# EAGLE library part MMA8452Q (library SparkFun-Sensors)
NXP MMA8452Q 3-Axis Digital Accelerometer The MMA8452Q is a smart low-power, three-axis, capacitive MEMS accelerometer with 12 bits of resolution. This accelerometer is packed with embedded functions with flexible user programmable options, configurable to two interrupt pins. Supply Voltage: 1.6-3.6V Range: +/- 2g, 4g, 8g Interface: I2C, 12-bit and 8-bit ODR: 1.56 Hz - 800 Hz Package: QFN-16 Datasheet SparkFun Products SparkFun Triple Axis Accelerometer Breakout - MMA8452Q (SEN-12756) SparkFun RedBot Sensor - Accelerometer (SEN-12589)
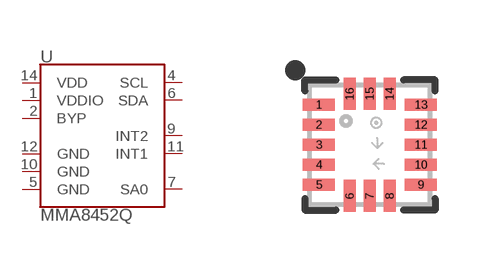
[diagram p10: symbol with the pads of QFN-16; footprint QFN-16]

Designator prefix U

## MMA8452Q (PROD_ID: IC-10769)  [QFN-16]
1  VDDIO
2  BYP
4  SCL
5  GND
6  SDA
7  SA0
9  INT2
10  GND
11  INT1
12  GND
14  VDD

## Footprint QFN-16 (pad centres in mm)
16-Pin Quad Flat No-Lead (QFN) (3 x 3 mm) Datasheet. Layout based on app note AN4077 Specifications: Pin Count: 16 Dimensions: 3.0 x 3.0 x 1.0 mm Pitch: 0.5 mm Devices Using: MMA8452Q
smd 0.8 x 0.3: 1 -1.275,1; 2 -1.275,0.5; 3 -1.275,0; 4 -1.275,-0.5; 5 -1.275,-1; 9 1.275,-1; 10 1.275,-0.5; 11 1.275,0; 12 1.275,0.5; 13 1.275,1
smd 0.3 x 0.8: 6 -0.5,-1.275; 7 0,-1.275; 8 0.5,-1.275; 14 0.5,1.275; 15 0,1.275; 16 -0.5,1.275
